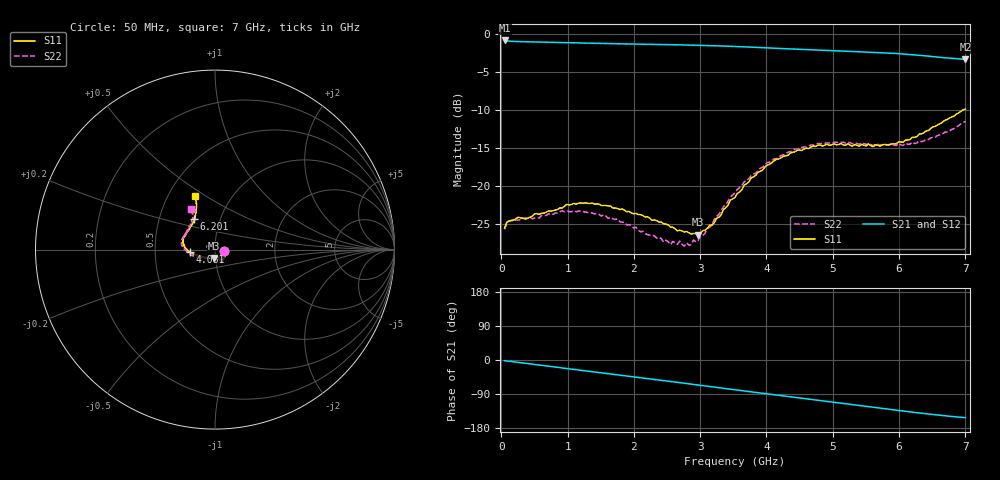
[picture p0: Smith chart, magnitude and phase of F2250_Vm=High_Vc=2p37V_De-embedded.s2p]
! Integrated Device Technology
! Corporate Headquarters
! 6024 Silver Creek Valley Road
! San Jose, CA 95138  USA
! Phone:  1-408-284-8200
! Toll Free:  1-800-223-1366
! Webpage:  http://www.idt.com/
! Timing and RF Division
! 515 Groton Road, Suite 102
! Westford, MA 01886-6024
! Device:  F2250
! Description: Voltage Variable RF Attenuator
! Frequency:  50.0 -  6000.00 MHz
! Package:  3x3 mm Thin QFN Plastic Package: 16 pin
! Ports:  2 RF, 3 DC
!  Pin  1  = GND
!  Pin  2  = NC
!  Pin  3  = RF1  = Port 1
!  Pin  4  = NC
!  Pin  5  = GND
!  Pin  6  = GND
!  Pin  7  = GND
!  Pin  8  = GND
!  Pin  9  = NC
!  Pin 10  = RF2  = Port 2
!  Pin 11  = NC
!  Pin 12  = GND
!  Pin 13  = GND
!  Pin 14  = VCNTRL
!  Pin 15  = VDD
!  Pin 16  = VMODE
! Vcntrl:  2.370 Volts
! Vmode:  +3.300 Volts
! Vdd:  +3.30  Volts
! Current:  1.313 mA
! Data:  The device was measured on a the F2250 evaluation board which has
!  individual transmission lines to the RF pins.  Data was collected
!  using a calibrated network analyzer.  The evaluation board was
!  de-embedded using a TRL calibration technique.
!  The reference plane is the edge of the package pin.
! Misc:  SN 10
!  Action Tracker AT0258
! Date Measured:  2014-11-26
! Date:  2015-10-15  MJV
! Note:
!  Integrated Device Technology supplies this data as a sample of measured
!  data at the package pin for this product.  Your particular data for this
!  product may vary.
!  Data was taken at 25 degrees C.
!  Integrated Device Technology reserves the right to change this data at anytime.
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# GHz S dB R 50
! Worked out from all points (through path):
!   201 points, 50 MHz to 7 GHz, reference 50 ohm
!   highest |S21| = -0.90 dB at 50 MHz (marker M1); lowest = -3.4 dB at 7 GHz (marker M2)
!   group delay of S21, straight-line fit = 61.2 ps
!   lowest |S11| = -26.4 dB at 2.969 GHz (marker M3), VSWR 1.10, Z = 49.2 - j4.66 ohm
!   |S11| at or under -10 dB: start of sweep to 6.971 GHz
!   |S22| runs from -28.0 to -11.6 dB; largest |S21 - S12| = 0.0019
!   S11 on the Smith chart (normalised r, x): 50 MHz: 1.11, -0.02; 4.081 GHz: 0.75, -0.02; 6.201 GHz: 0.75, +0.27; 7 GHz: 0.68, +0.45
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0.05  -25.58 -10.6  -0.90 -1.8  -0.90 -1.8  -25.74 -10.8
0.1195  -24.67 -10.1  -0.99 -3.2  -0.99 -3.2  -24.61 -8.8
0.57125  -23.77 -31.2  -1.11 -13.3  -1.10 -13.3  -24.26 -31.3
0.91875  -22.94 -49.9  -1.18 -21.0  -1.18 -21.1  -23.29 -50.9
1.2315  -22.31 -57.6  -1.24 -27.9  -1.24 -27.9  -23.41 -61.4
1.75275  -22.98 -64.6  -1.33 -39.1  -1.33 -39.1  -24.36 -67.8
2.37825  -24.79 -64.3  -1.43 -52.8  -1.43 -52.8  -26.78 -67.0
2.552  -25.44 -69.2  -1.45 -56.7  -1.45 -56.7  -27.76 -73.3
2.691  -25.85 -77.2  -1.48 -59.8  -1.48 -59.8  -27.28 -81.1
2.7605  -26.09 -79.4  -1.49 -61.3  -1.49 -61.3  -27.95 -85.5
2.969  -26.43 -97.4  -1.53 -66.0  -1.53 -66.0  -27.20 -105.0
3.1775  -25.19 -120.4  -1.58 -70.7  -1.58 -70.7  -25.18 -126.7
3.525  -21.54 -152.4  -1.69 -78.5  -1.68 -78.6  -20.93 -148.7
3.76825  -18.98 -164.5  -1.78 -84.0  -1.78 -84.1  -18.67 -159.6
4.081  -16.96 -175.5  -1.90 -91.0  -1.90 -91.0  -16.70 -171.4
4.4285  -15.55 176.1  -2.03 -98.6  -2.04 -98.7  -15.19 178.7
4.7065  -14.77 169.2  -2.13 -104.8  -2.14 -104.8  -14.68 173.0
5.054  -14.62 161.0  -2.26 -112.5  -2.26 -112.5  -14.27 165.9
5.85325  -14.58 135.2  -2.56 -130.0  -2.56 -130.1  -14.68 147.2
6.20075  -13.63 123.7  -2.77 -137.7  -2.77 -137.8  -14.26 138.2
6.54825  -12.20 115.7  -3.04 -144.7  -3.05 -144.9  -13.59 126.9
7  -9.92 110.8  -3.37 -152.1  -3.38 -152.2  -11.55 120.6
